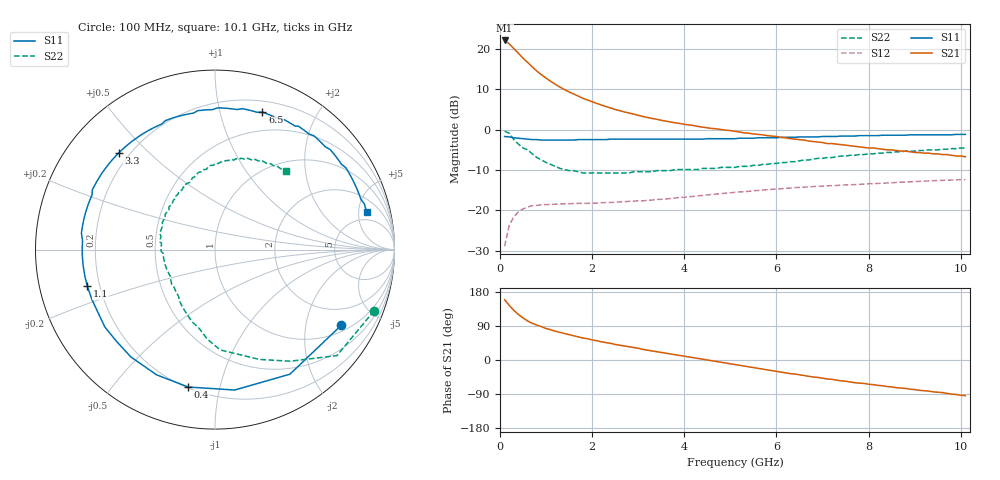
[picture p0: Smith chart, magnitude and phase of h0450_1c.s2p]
!HBFP-0450
!S and NOISE PARAMETERS at Vce=1V  Ic=5mA.  LAST UPDATED  09-04-98
# GHZ S MA R  50
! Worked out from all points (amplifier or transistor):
!   101 points, 100 MHz to 10.1 GHz, reference 50 ohm
!   highest |S21| = 22.0 dB at 100 MHz (marker M1)
!   |S21| within 3 dB of that: start of sweep to 384.4 MHz
!   unconditionally stable (mu >= 1): 2.971 GHz to end of sweep
!   at 1.7 GHz: K = 0.62, MSG = 13.3 dB, |S12| = -18.3 dB
!   at 5.1 GHz: K = 1.26, MAG = 4.5 dB, |S12| = -15.5 dB
!   at 10.1 GHz: K = 1.14, MAG = 0.6 dB, |S12| = -12.4 dB
!   lowest NFmin = 1.17 dB at 1.8 GHz
!   S11 on the Smith chart (normalised r, x): 100 MHz: 1.23, -3.17; 400 MHz: 0.21, -0.80; 1.1 GHz: 0.15, -0.14; 3.3 GHz: 0.16, +0.41; 6.5 GHz: 0.30, +1.36; 10.1 GHz: 3.54, +6.14
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0.1  0.82 -31.0  12.65 159.0  0.036 73.0  0.95 -21.0
0.2  0.81 -59.0  11.47 144.0  0.065 57.0  0.9 -41.0
0.3  0.79 -82.0  10.03 131.0  0.083 47.0  0.75 -56.0
0.4  0.78 -101.0  8.77 120.0  0.096 39.0  0.66 -68.0
0.5  0.77 -115.0  7.62 111.0  0.104 32.0  0.59 -79.0
0.6  0.76 -128.0  6.77 103.0  0.11 27.0  0.56 -87.0
0.7  0.75 -137.0  5.95 97.0  0.114 23.0  0.5 -95.0
0.8  0.75 -145.0  5.28 92.0  0.115 20.0  0.45 -101.0
1  0.74 -158.0  4.32 83.0  0.118 16.0  0.39 -114.0
1.1  0.74 -164.0  3.95 80.0  0.118 14.0  0.37 -119.0
1.2  0.74 -168.0  3.63 76.0  0.119 12.0  0.35 -124.0
1.4  0.74 -177.0  3.12 70.0  0.12 10.0  0.32 -133.0
1.8  0.75 170.0  2.43 58.0  0.122 7.0  0.29 -149.0
2.2  0.75 158.0  2.01 48.0  0.124 5.0  0.29 -162.0
2.5  0.76 152.0  1.77 41.0  0.126 4.0  0.29 -169.0
3.3  0.76 135.0  1.37 24.0  0.134 1.0  0.3 173.0
3.5  0.76 131.0  1.3 20.0  0.137 0.0  0.31 170.0
5.1  0.77 99.0  0.95 -12.0  0.167 -10.0  0.34 139.0
6.5  0.81 71.0  0.75 -39.0  0.192 -25.0  0.41 109.0
6.8  0.81 66.0  0.71 -45.0  0.197 -28.0  0.43 104.0
8.5  0.85 38.0  0.56 -71.0  0.219 -47.0  0.52 75.0
10.1  0.87 14.0  0.46 -94.0  0.239 -69.0  0.59 48.0
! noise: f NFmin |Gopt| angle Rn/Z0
1.8  1.17  0.56  166  0.04
2  1.24  0.56  175  0.04
2.5  1.42  0.59  -168  0.05
3.5  1.74  0.67  -142  0.16
4  2  0.7  -129  0.29
5  2.34  0.74  -106  0.71
5.5  2.47  0.77  -94  1.06
7  3  0.81  -64  2.48
8  3.33  0.83  -47  3.71
10  4.03  0.82  -16  5.96
